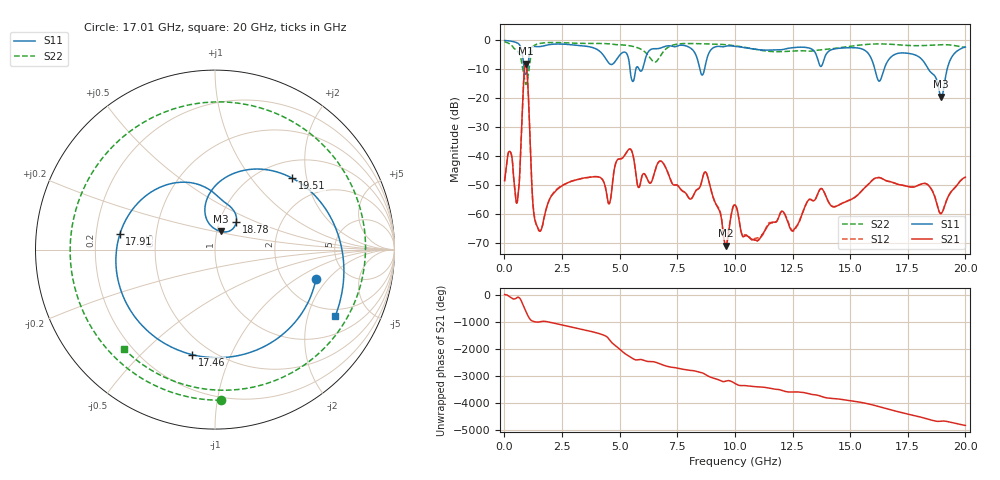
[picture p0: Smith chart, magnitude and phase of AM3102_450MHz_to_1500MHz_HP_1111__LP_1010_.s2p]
!Agilent Technologies,E8364B,MY43040894,A.07.50.67
!Agilent E8364B: A.07.50.67
!Date: Thursday, January 11, 2018 06:51:08
!Correction: S11(Full 2 Port(1,2))
!S21(Full 2 Port(1,2))
!S12(Full 2 Port(1,2))
!S22(Full 2 Port(1,2))
!S2P File: Measurements: S11, S21, S12, S22:
# Hz S  dB  R 50
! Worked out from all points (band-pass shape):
!   1601 points, 10 MHz to 20 GHz, reference 50 ohm
!   highest |S21| = -8.03 dB at 922 MHz (marker M1); lowest = -71.0 dB at 9.605 GHz (marker M2)
!   |S21| within 3 dB of the highest: 860.3 MHz to 983.9 MHz (123.6 MHz wide, 13.4 % of centre)
!   lowest |S11| = -19.5 dB at 18.95 GHz (marker M3), VSWR 1.24, Z = 52.1 + j10.7 ohm
!   |S11| at or under -10 dB: 5.451 GHz to 5.701 GHz (250.2 MHz wide, 4.49 % of centre); 16.07 GHz to 16.47 GHz (398.7 MHz wide, 2.45 % of centre); 18.4 GHz to 19.21 GHz (810.8 MHz wide, 4.31 % of centre)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
!   |S22| runs from -15.2 to -0.5 dB; largest |S21 - S12| = 0.00091
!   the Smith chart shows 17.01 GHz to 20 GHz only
!   S11 on the Smith chart (normalised r, x): 17.01 GHz: 3.00, -1.51; 17.46 GHz: 0.40, -0.73; 17.91 GHz: 0.30, +0.07; 18.78 GHz: 1.20, +0.38; 19.51 GHz: 1.36, +1.65; 20 GHz: 1.68, -3.02
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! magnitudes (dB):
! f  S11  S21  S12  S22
! 10 MHz  -0.1  -48.5  -48.6  -0.5
! 572.2 MHz  -1.0  -55.2  -55.1  -3.7
! 922 MHz  -11.8  -8.0  -8.0  -15.1
! 1.247 GHz  -2.1  -57.4  -57.1  -2.3
! 1.447 GHz  -2.2  -64.7  -64.7  -1.2
! 3.346 GHz  -1.9  -47.7  -47.8  -1.1
! 4.545 GHz  -8.0  -56.4  -56.5  -1.2
! 5.57 GHz  -14.2  -39.3  -39.4  -2.1
! 6.682 GHz  -2.9  -42.1  -42.2  -6.5
! 8.756 GHz  -7.3  -45.7  -45.8  -1.2
! 9.605 GHz  -2.0  -71.0  -71.0  -1.5
! 10.01 GHz  -2.1  -56.9  -56.9  -1.9
! 10.93 GHz  -3.2  -69.1  -68.4  -3.2
! 13.34 GHz  -3.1  -55.3  -55.3  -3.7
! 16.68 GHz  -6.6  -48.8  -48.7  -1.3
! 17.01 GHz  -4.6  -49.7  -49.6  -1.5
! 17.46 GHz  -4.5  -50.4  -50.5  -1.8
! 17.91 GHz  -5.4  -50.3  -50.2  -1.9
! 18.78 GHz  -14.2  -57.0  -56.9  -1.6
! 18.95 GHz  -19.5  -59.8  -59.9  -1.5
! 19.51 GHz  -4.6  -51.2  -51.1  -1.8
! 20 GHz  -2.3  -47.3  -47.4  -2.5
